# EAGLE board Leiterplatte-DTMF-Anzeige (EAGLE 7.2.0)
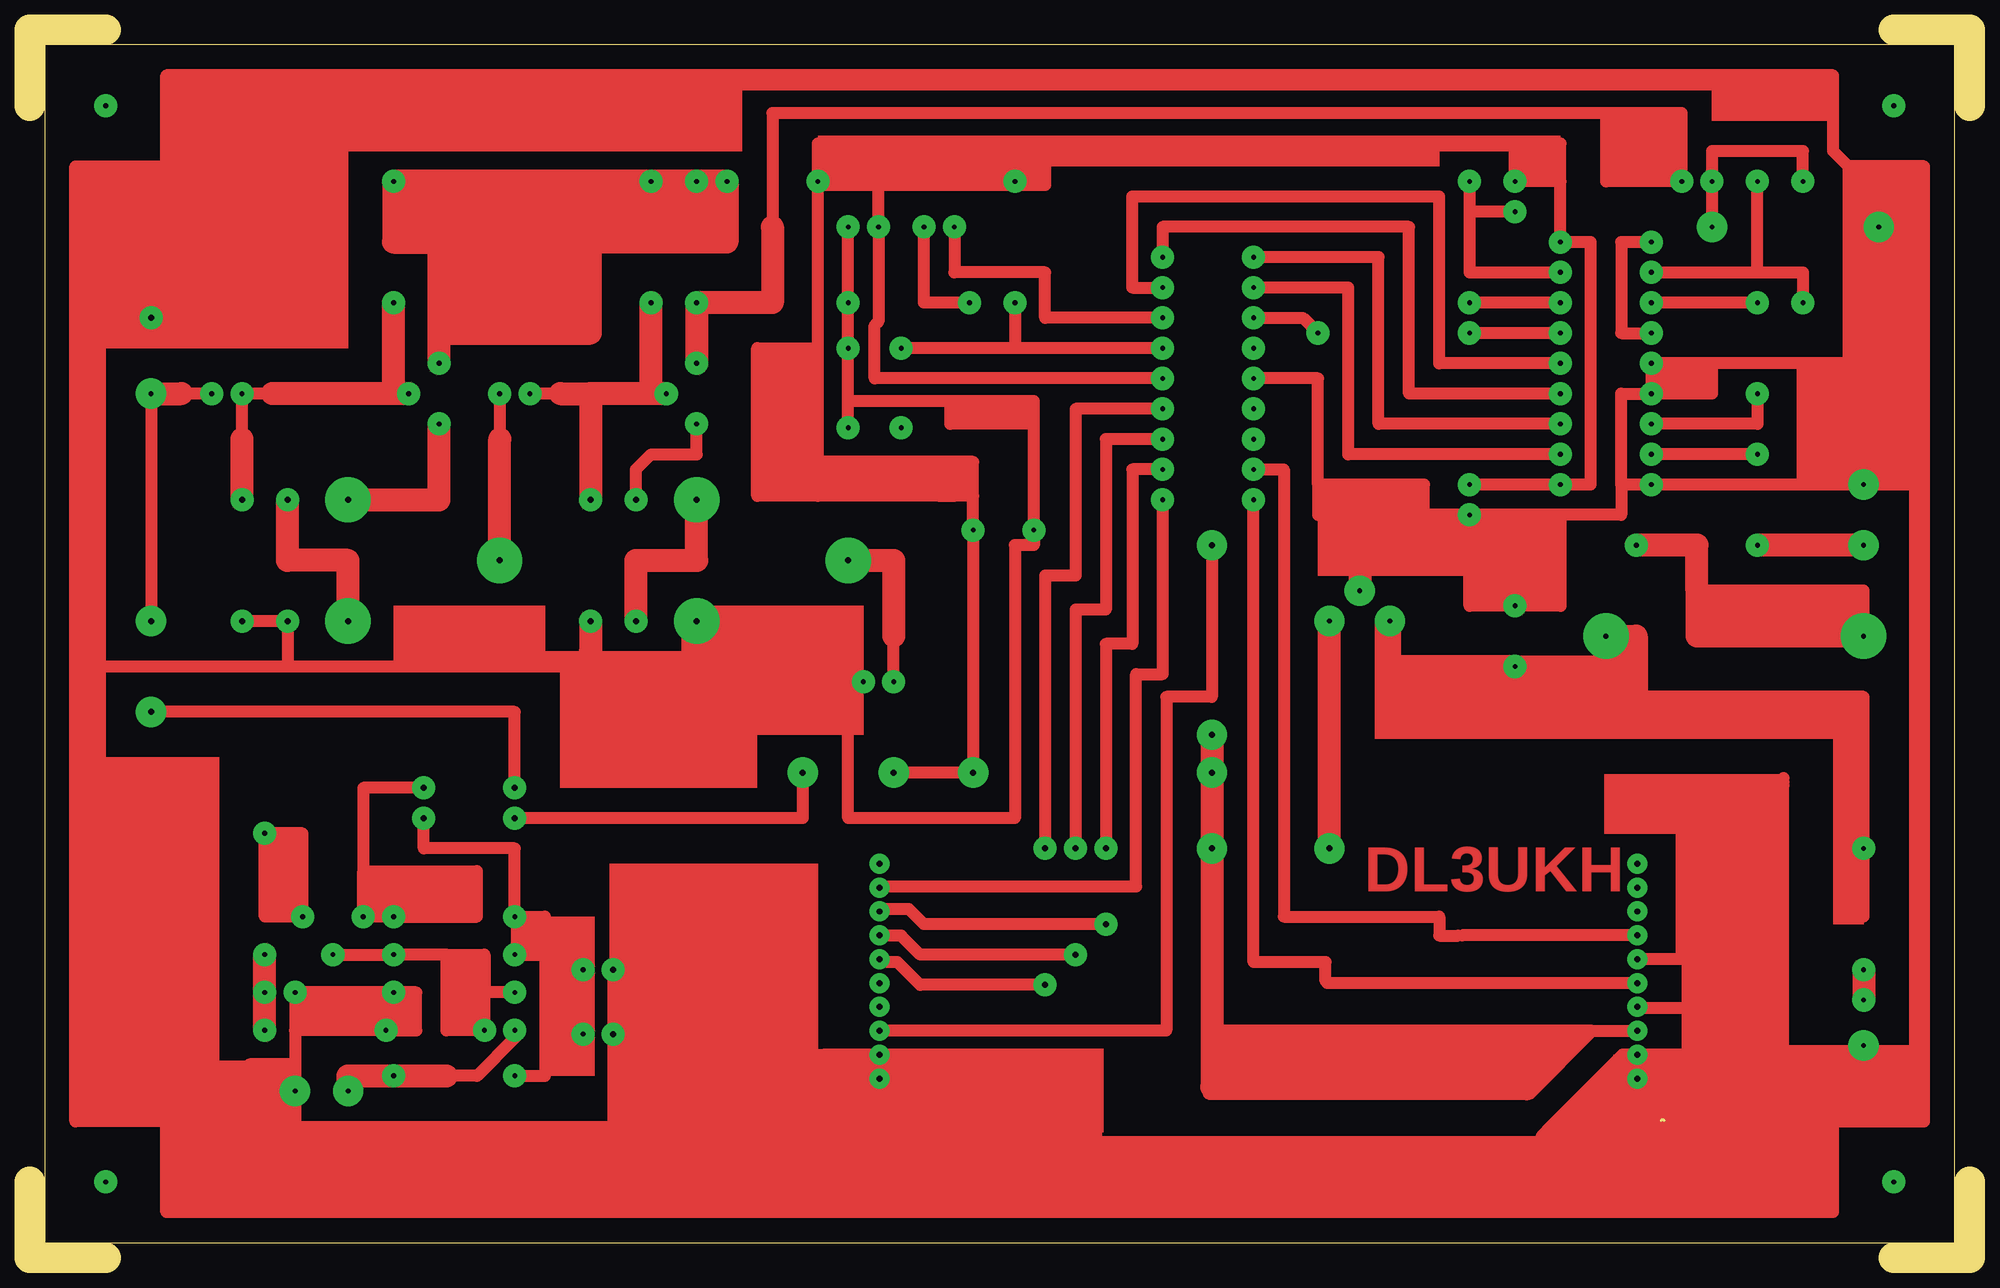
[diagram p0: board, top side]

Size 162.56 x 102.87 mm. Coordinates in mm from the lower left corner, seen from the top.
Outline: 0,96.52 0,102.87 6.35,102.87
Outline: 0,6.35 0,0 6.35,0
Outline: 156.21,0 162.56,0 162.56,6.35
Outline: 162.56,96.52 162.56,102.87 156.21,102.87
Outline: 136.95,11.5 136.7,11.5
Outline: 1.27,101.6 1.27,1.27 161.29,1.27 161.29,101.6 1.27,101.6
Copper layers (1*16): Top 0.035mm / dielectric 1.5mm / Bottom 0.035mm
Design rules "default": minimum track width 10mil, minimum drill 24mil, track to track 8mil, track to pad 8mil, pad to pad 8mil, via to via 8mil, smd to smd 8mil, copper to edge 40mil, drill to drill 8mil, minimum pad ring 10mil, minimum via ring 8mil, stop-mask expansion 4mil, vias tented up to drill 0mil, thermal gap 10mil

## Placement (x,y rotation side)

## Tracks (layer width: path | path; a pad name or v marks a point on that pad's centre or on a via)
S$1  (via drill 0.4 pad 1.93)
  other vias: 6.35,6.35
S$2  (via drill 0.4 pad 1.93)
  other vias: 6.35,96.52
S$3  (via drill 0.4 pad 1.93)
  other vias: 156.21,6.35
S$4  (via drill 0.4 pad 1.93)
  other vias: 156.21,96.52
S$5  (via drill 0.4 pad 1.93)
  other vias: 55.88,90.17
S$6  (via drill 0.4 pad 1.93)
  Top 1.016: v94.93,81.28 92.39,81.28 92.39,88.9 118.11,88.9 118.11,74.93 v128.27,74.93
S$7  (via drill 0.4 pad 1.93)
  Top 1.016: v82.55,90.17 81.28,93.03
S$8  (via drill 0.4 pad 1.93)
  Top 1.016: v94.93,76.2 82.55,76.2 | v82.55,80.01 82.55,76.2 | 82.55,76.2 v73.02,76.2 | v78.74,80.01 74.93,80.01 v74.93,86.36 | v94.93,78.74 85.09,78.74 85.09,82.55 77.47,82.55 v77.47,86.36
S$9  (via drill 0.4 pad 1.93)
  Top 1.016: 71.12,93.34 v71.12,86.36 71.12,78.42 70.8,78.1 70.8,73.66 v94.93,73.66
S$10  (via drill 0.4 pad 1.93, 0.4 pad 2.54)
  Top 1.016: v102.55,73.66 107.95,73.66 107.95,64.77 | 107.95,64.77 107.95,62.23 114.3,62.23 | 107.95,64.77 116.84,64.77 116.84,62.23 | 114.3,62.23 111.44,58.74 | 116.84,62.23 114.3,62.23 | v120.65,62.23 116.84,62.23 | v120.65,62.23 120.65,54.61 128.27,54.61 128.27,62.23 | 124.46,62.23 v120.65,62.23 | 124.46,62.23 124.46,58.42 | 128.27,62.23 124.46,62.23 | 128.27,62.23 133.35,62.23 133.35,64.77 | v135.89,72.39 133.35,72.39 133.35,64.77 | v135.89,72.39 140.97,72.39 140.97,74.93 | v135.89,72.39 v135.89,74.93 140.97,74.93 | 133.35,64.77 v135.89,64.77 148.59,64.77 | 148.59,64.77 148.59,74.93 | 152.4,74.93 148.59,74.93 | 152.4,74.93 154.94,74.93 | 148.59,74.93 140.97,74.93 | 152.4,91.44 151.13,92.71 151.13,99.06 11.43,99.06 11.43,91.44 3.81,91.44 3.81,50.8 | 152.4,91.44 152.4,74.93 | 152.4,64.77 148.59,64.77 | 152.4,64.77 152.4,74.93 | 152.4,64.77 v153.67,64.77 158.75,64.77 | 152.4,91.44 158.75,91.44 158.75,64.77 | 3.81,50.8 5.08,50.8 | 3.81,50.8 3.81,11.43 11.43,11.43 11.43,3.81 151.13,3.81 151.13,11.43 158.75,11.43 158.75,64.77
  Top 1.93: 111.44,58.74 v111.44,55.88 | 124.46,58.42 v124.46,54.61
S$11  (via drill 0.4 pad 1.93)
  other vias: 73.02,69.53
S$12  (via drill 0.4 pad 1.93)
  other vias: 102.55,68.58
S$13  (via drill 0.4 pad 1.93)
  other vias: 102.55,71.12
S$14  (via drill 0.4 pad 1.93)
  Top 1.016: 62.23,86.36 62.23,95.88 132.08,95.88 | 132.08,95.88 138.43,95.88 v138.43,90.17 132.08,90.17 132.08,95.88
  Top 1.93: v55.88,74.93 v55.88,80.01 62.23,80.01 62.23,86.36
S$15  (via drill 0.4 pad 1.93)
  Top 1.016: v68.58,86.36 v68.58,80.01 68.58,71.75 | v68.58,69.53 68.58,71.75 | 77.15,71.75 84.14,71.75 84.14,69.85 | 77.15,71.75 68.58,71.75 | 84.14,69.85 v84.14,60.96 84.14,59.69 82.55,59.69 82.55,36.83 68.58,36.83 68.58,44.45 | 84.14,69.85 77.15,69.85 77.15,71.75
S$16  (via drill 0.4 pad 2.54)
  other vias: 154.94,86.36
S$17  (via drill 0.4 pad 1.93)
  other vias: 68.58,76.2
S$18  (via drill 0.4 pad 1.93, 0.4 pad 3.81)
  Top 1.016: v153.67,52.07 153.67,55.88 139.7,55.88
  Top 1.93: v153.67,52.07 139.7,52.07 139.7,55.88 139.7,59.69 v134.62,59.69
S$19  (via drill 0.4 pad 1.93)
  Top 1.93: v153.67,24.13 v153.67,21.59
S$20  (via drill 0.5 pad 1.93)
  other vias: 10.16,78.74
S$21  (via drill 0.4 pad 1.93, 0.4 pad 2.54)
  Top 1.93: v153.67,59.69 v144.78,59.69
S$22  (via drill 0.4 pad 2.54)
  Top 1.93: 108.9,34.29 v108.9,53.34
S$23
  Top 1.016: 134.62,20.95 139.38,20.95
S$24  (via drill 0.4 pad 1.93, 0.4 pad 2.54)
  Top 1.016: v29.84,19.05 30.48,19.05 v30.48,22.22 | v30.48,22.22 v22.22,22.22 22.22,19.05 | v29.84,19.05 32.38,19.05 32.38,22.22 v30.48,22.22 | 22.22,19.05 v22.22,13.97 | v29.84,19.05 22.22,19.05 | v22.22,13.97 22.22,11.43 | 22.22,11.43 22.22,10.16 | 22.22,11.43 18.41,11.43 | 18.41,11.43 18.41,10.16 21.91,10.16 | v22.22,13.97 22.22,16.19 18.41,16.19 18.41,11.43
S$25  (via drill 0.4 pad 1.93)
  other vias: 102.55,66.04
S$26  (via drill 0.5 pad 1.93, 0.5 pad 2.54)
  Top 1.016: v40.64,39.37 40.64,45.72 v10.16,45.72
S$27  (via drill 0.5 pad 1.68)
  other vias: 134.7,21
S$28  (via drill 0.5 pad 1.68)
  Top 1.016: v134.7,31 134.75,31 134.75,31.06
S$29  (via drill 0.4 pad 1.93)
  Top 1.016: 124.46,93.34 v124.46,90.17 128.27,90.17 | 128.27,90.17 128.27,93.34 | 128.27,90.17 v128.27,85.09 130.81,85.09 130.81,64.77 v128.27,64.77 v120.65,64.77
S$30  (via drill 0.5 pad 1.68)
  Top 1.016: 71.35,31.07 71.35,31 v71.2,31
S$31  (via drill 0.5 pad 1.68)
  Top 1.016: 71.39,28.85 71.39,29 v71.2,29
S$32  (via drill 0.4 pad 1.93, 0.4 pad 2.54, 0.5 pad 2.54)
  Top 1.016: v15.24,72.39 12.7,72.39 | v10.16,72.39 v10.16,53.34
  Top 1.93: v10.16,72.39 12.7,72.39
S$33  (via drill 0.4 pad 1.93, 0.5 pad 1.93)
  Top 1.016: v94.93,66.04 92.39,66.04 92.39,51.44 90.17,51.44 v90.17,34.29
S$34  (via drill 0.4 pad 1.93, 0.5 pad 1.93)
  Top 1.016: v94.93,68.58 90.17,68.58 90.17,54.29 87.63,54.29 v87.63,34.29
S$35  (via drill 0.4 pad 1.93, 0.5 pad 1.93)
  Top 1.016: v94.93,71.12 87.63,71.12 87.63,57.15 85.09,57.15 v85.09,34.29
S$36  (via drill 0.4 pad 2.54)
  other vias: 153.67,17.78
S$37  (via drill 0.5 pad 1.68)
  Top 1.016: 71.11,26.94 71.11,27 v71.2,27
S$38  (via drill 0.5 pad 1.68)
  Top 1.016: 71.15,25.04 71.15,25 v71.2,25
S$39  (via drill 0.4 pad 1.93, 0.5 pad 3.81)
  Top 1.016: v39.37,72.39 39.37,68.58
  Top 1.93: v39.37,58.42 39.37,68.58
S$40  (via drill 0.5 pad 1.68)
  Top 1.016: 71.17,33.03 71.17,32.93 71.2,32.93 v71.2,33.01
S$41
  Top 1.016: 102.55,66.04 105.09,66.04 105.09,28.57 118.11,28.57 118.11,26.99 119.7,26.99
S$42  (via drill 0.4 pad 1.93, 0.5 pad 1.93)
  Top 1.016: v50.8,63.5 50.8,66.04 52.07,67.31 55.88,67.31 v55.88,69.85
S$43  (via drill 0.5 pad 1.93, 0.5 pad 3.81)
  Top 1.93: v50.8,53.34 50.8,58.42 55.88,58.42 v55.88,63.5
S$44  (via drill 0.4 pad 1.93, 0.5 pad 1.93, 0.5 pad 3.81)
  Top 1.016: v69.85,48.26 67.31,48.26 66.04,49.53 55.88,49.53 | 55.88,50.8 55.88,49.53 | v17.78,53.34 v21.59,53.34 21.59,49.53 | 46.99,50.8 46.99,49.53 | 46.99,49.53 21.59,49.53 | 21.59,49.53 6.35,49.53 | 55.88,49.53 46.99,49.53
  Top 1.93: v55.88,53.34 55.88,50.8 | v46.99,53.34 46.99,50.8
S$45  (via drill 0.4 pad 1.93, 0.5 pad 3.81)
  Top 1.016: v72.39,48.26 72.39,52.07
  Top 1.93: v68.58,58.42 72.39,58.42 72.39,52.07
S$46  (via drill 0.4 pad 1.93, 0.5 pad 1.93)
  Top 1.016: 44.45,72.39 v41.91,72.39
  Top 1.93: v52.07,80.01 52.07,72.39 v53.34,72.39 46.99,72.39 | 44.45,72.39 46.99,72.39 | 46.99,72.39 v46.99,63.5
S$47  (via drill 0.5 pad 1.68)
  Top 1.016: 134.79,29.16 134.79,29 v134.7,29
S$48  (via drill 0.5 pad 1.68)
  Top 1.016: 109.29,16.15 109.29,16.25 98.77,13.75 125.7,13.75 130.95,19 v134.7,19
S$49  (via drill 0.5 pad 1.68)
  Top 1.016: 70.98,19.09 70.98,19 v71.2,19
S$50  (via drill 0.4 pad 1.93)
  Top 1.016: v135.89,82.55 144.78,82.55 | 144.78,82.55 v144.78,90.17 | 144.78,82.55 148.59,82.55 v148.59,80.01
S$51  (via drill 0.4 pad 1.93)
  Top 1.016: v135.89,85.09 133.35,85.09 133.35,77.47 v135.89,77.47
S$52  (via drill 0.4 pad 1.93, 0.5 pad 3.81)
  Top 1.93: v26.67,63.5 34.29,63.5 v34.29,69.85
S$53  (via drill 0.5 pad 1.68)
  other vias: 134.7,15
S$54  (via drill 0.5 pad 1.68)
  Top 1.016: v71.2,15 67.34,15
S$55  (via drill 0.5 pad 1.68)
  Top 1.016: v134.7,33.01 134.39,33.01 134.39,32.97
S$56  (via drill 0.5 pad 1.93, 0.5 pad 3.81)
  Top 1.93: v26.67,53.34 26.67,58.42 21.59,58.42 v21.59,63.5
S$59
  Top 1.016: 147,10.48 147,9.84 126.68,9.84 | 126.68,9.84 126.68,10.16 128.91,12.38 | 126.68,9.84 126.68,4.13
S$60  (via drill 0.5 pad 2.54)
  other vias: 108.9,34.29
S$61  (via drill 0.5 pad 2.54)
  Top 1.93: v99.06,43.82 v99.06,40.64 v99.06,34.29 99.06,14.29
S$62
  Top 1.016: 125.41,13.65 125.41,13.97
S$63  (via drill 0.5 pad 1.68)
  other vias: 134.7,21
S$64  (via drill 0.5 pad 1.68)
  other vias: 134.7,25
S$65  (via drill 0.5 pad 1.68)
  Top 1.016: v71.2,17 67.34,17
S$66  (via drill 0.5 pad 1.68)
  other vias: 71.2,21
S$67  (via drill 0.5 pad 1.68)
  other vias: 71.2,23
S$68  (via drill 0.4 pad 1.93, 0.5 pad 1.93)
  Top 1.016: 20.32,72.39 v17.78,72.39 17.78,68.58
  Top 1.93: 30.48,72.39 v30.48,80.01 | 30.48,72.39 20.32,72.39 | v31.75,72.39 30.48,72.39 | v17.78,63.5 17.78,68.58
S$69  (via drill 0.5 pad 1.68)
  Top 1.016: v134.7,31 134.75,31 134.75,31.06
S$70  (via drill 0.5 pad 1.68)
  Top 1.016: 71.03,31.07 71.35,31 v71.2,31
S$71  (via drill 0.5 pad 1.68)
  Top 1.016: 71.07,28.85 71.07,29 v71.2,29
S$72  (via drill 0.5 pad 1.68)
  Top 1.016: 71.11,26.94 71.11,27 v71.2,27
S$73  (via drill 0.5 pad 1.68)
  Top 1.016: 71.15,25.04 71.15,25 v71.2,25
S$74  (via drill 0.5 pad 1.68)
  Top 1.016: 71.17,33.03 71.17,32.93 71.2,32.93 v71.2,33.01
S$75  (via drill 0.5 pad 1.68)
  Top 1.016: 134.79,29.16 134.79,29 v134.7,29
S$76  (via drill 0.5 pad 1.68)
  Top 1.016: 109.29,16.15 109.29,16.25 103.85,13.75 109.45,13.75 | 109.45,13.75 125.7,13.75 130.95,19 | 130.95,19 v134.7,19 | 130.95,19 109.45,19 109.45,13.75
S$77  (via drill 0.5 pad 1.68)
  Top 1.016: 71.3,19.09 71.3,19 v71.2,19
S$78  (via drill 0.5 pad 1.68)
  Top 1.016: v71.2,15 67.34,15
S$79  (via drill 0.5 pad 1.68)
  Top 1.016: v134.7,33.01 v134.71,33.01 134.71,32.97
S$82  (via drill 0.5 pad 1.68)
  other vias: 134.7,23
S$83  (via drill 0.5 pad 1.68)
  other vias: 134.7,23 134.7,23
S$84  (via drill 0.5 pad 1.68)
  other vias: 134.7,27
S$85  (via drill 0.5 pad 2.54)
  Top 1.016: v99.06,59.69 99.06,46.99 95.25,46.99 95.25,19.05 71.12,19.05
S$86  (via drill 0.4 pad 1.93)
  Top 1.016: 71.12,31.11 92.71,31.11 92.71,48.9 94.93,48.9 v94.93,63.5
S$87  (via drill 0.5 pad 1.93)
  Top 1.016: v90.17,27.94 74.93,27.94 73.66,29.21 71.12,29.21
S$88  (via drill 0.5 pad 1.93)
  Top 1.016: v48.89,24.13 48.89,4.13
S$89  (via drill 0.4 pad 1.68)
  Top 1.016: v134.7,25 134.73,25 134.73,25.34 134.83,25.03
  other vias: 134.7,21
S$90  (via drill 0.4 pad 1.68)
  Top 1.016: v71.2,17 67.97,17
S$91  (via drill 0.4 pad 1.68)
  other vias: 71.2,21
S$92  (via drill 0.4 pad 1.68)
  other vias: 71.2,23
S$93  (via drill 0.4 pad 1.68)
  Top 1.016: v134.7,31 134.75,31 134.75,31.06
S$94  (via drill 0.4 pad 1.68)
  Top 1.016: 71.03,31.07 71.35,31 v71.2,31
S$95  (via drill 0.4 pad 1.68)
  Top 1.016: 71.39,28.85 71.39,29 v71.2,29
S$96  (via drill 0.4 pad 1.68)
  Top 1.016: 71.11,26.94 71.11,27 v71.2,27
S$97  (via drill 0.4 pad 1.68)
  Top 1.016: 71.15,25.04 71.47,25 v71.2,25
S$98  (via drill 0.4 pad 1.68)
  Top 1.016: 71.17,33.03 71.17,32.93 71.2,32.93 v71.2,33.01
S$99  (via drill 0.4 pad 1.68)
  Top 1.016: 134.79,29.16 134.79,29 v134.7,29
S$100  (via drill 0.4 pad 1.68)
  Top 1.016: 109.29,16.15 109.61,16.25 102.58,13.75 109.45,13.75 | 109.45,13.75 125.7,13.75 130.95,19 | 130.95,19 v134.7,19 | 130.95,19 109.45,19 109.45,13.75
S$101  (via drill 0.4 pad 1.93)
  Top 1.93: 34.29,90.17 v52.07,90.17 v58.42,90.17 58.42,85.09 35.56,85.09 34.29,85.09 | 34.29,90.17 v30.48,90.17 30.48,85.09 34.29,85.09 | v34.29,74.93 34.29,77.47 | 34.29,77.47 34.29,85.09 | 34.29,85.09 34.29,90.17 | 34.29,77.47 46.99,77.47 46.99,86.36
S$102  (via drill 0.4 pad 1.93)
  Top 1.016: v128.27,80.01 v120.65,80.01
S$103  (via drill 0.4 pad 1.93)
  Top 1.016: v128.27,77.47 v120.65,77.47
S$104  (via drill 0.4 pad 1.68)
  Top 1.016: 71.3,19.09 71.3,19 v71.2,19
S$105  (via drill 0.4 pad 1.93)
  Top 1.016: v128.27,72.39 115.57,72.39 115.57,86.36 94.93,86.36 v94.93,83.82
S$106  (via drill 0.4 pad 1.93)
  Top 1.016: v128.27,69.85 113.03,69.85 113.03,83.82 v102.55,83.82
S$107  (via drill 0.4 pad 1.93)
  Top 1.016: v128.27,67.31 110.49,67.31 110.49,81.28 v102.55,81.28
S$108  (via drill 0.4 pad 1.93)
  Top 1.016: v102.55,78.74 106.68,78.74 v107.95,77.47
S$109  (via drill 0.4 pad 1.68)
  Top 1.016: v71.2,15 67.34,15
S$110  (via drill 0.4 pad 1.93)
  other vias: 102.55,76.2
S$111  (via drill 0.4 pad 1.68)
  Top 1.016: v134.7,33.01 v134.71,33.01 134.71,32.97
S$113  (via drill 0.4 pad 1.68)
  Top 1.016: v134.7,23 108.7,23 108.7,23.12
S$114  (via drill 0.4 pad 1.68)
  Top 1.016: v134.7,23 126.45,23
S$115  (via drill 0.4 pad 1.93)
  Top 1.016: v120.65,90.17 120.65,87.63 | 120.65,87.63 120.65,82.55 v128.27,82.55 | v124.46,87.63 120.65,87.63
S$116  (via drill 0.4 pad 1.68)
  Top 1.016: v134.7,27 120.02,27
S$117  (via drill 0.4 pad 1.93)
  Top 1.016: 46.35,26.99 v46.35,24.13 v46.35,18.73 | 46.35,15.88 v46.35,18.73 | v46.35,18.73 46.35,25.4
S$118  (via drill 0.4 pad 1.93)
  Top 1.016: v144.78,67.31 v135.89,67.31
S$119  (via drill 0.4 pad 1.93)
  Top 1.016: v144.78,72.39 144.78,69.85 v135.89,69.85
S$120  (via drill 0.4 pad 1.93)
  Top 1.016: v144.78,80.01 v135.89,80.01
S$121  (via drill 0.4 pad 1.68)
  Top 1.016: 128.45,11 132.45,15 v134.7,15 v134.7,17 133.45,17 127.2,10.75
S$123  (via drill 0.4 pad 1.93, 0.4 pad 2.54)
  Top 1.016: v148.59,90.17 148.59,92.71 140.97,92.71 v140.97,90.17 v140.97,86.36
S$124  (via drill 0.5 pad 1.68)
  Top 1.016: 128.45,11 132.45,15 v134.7,15 v134.7,17 133.45,17 127.2,10.75
S$125  (via drill 0.5 pad 1.93)
  Top 1.016: v87.63,25.4 74.61,25.4 73.02,26.99 71.12,26.99
S$126  (via drill 0.5 pad 1.93)
  Top 1.016: v85.09,22.86 74.61,22.86 72.71,24.77 71.12,24.77
S$127  (via drill 0.4 pad 1.93)
  Top 1.016: 66.04,93.34 v66.04,90.17 66.04,89.85 | 66.04,76.2 66.04,89.85 | 66.04,63.82 66.04,66.67 | 66.04,66.67 66.04,76.2 | 66.04,76.2 60.96,76.2 60.96,63.82 76.2,63.82 | 76.2,63.82 77.47,63.82 | 85.09,91.44 85.09,89.85 66.04,89.85 | 76.2,63.82 76.2,66.67 | 76.2,66.67 66.04,66.67 | 77.47,63.82 77.47,66.67 | 77.47,66.67 76.2,66.67 | 79.06,63.82 v79.06,60.96 79.06,40.64 | 79.06,63.82 77.47,63.82 | 79.06,63.82 79.06,66.67 77.47,66.67
S$128  (via drill 0.5 pad 2.54)
  Top 1.016: v79.06,40.64 v72.39,40.64
S$129  (via drill 0.4 pad 1.68)
  Top 1.016: 134.63,21 v134.7,21 | 146.7,25 145.95,25 | 145.95,25 134.73,25 | v134.7,25 134.73,25 | 134.73,25 134.73,25.03 134.83,25.03 | 128.45,11 132.45,15 v134.7,15 | 127.2,10.75 133.45,17 v134.7,17 | v134.7,15 139.7,15 | v134.7,17 v134.7,15 | 138.95,17 v134.7,17 | 138.95,17 145.95,17 | 145.95,17 146.45,17 | 138.95,10.39 138.95,17 | 145.95,25 145.95,17
S$130  (via drill 0.4 pad 1.93, 0.4 pad 2.54, 0.4 pad 3.81)
  Top 1.016: v124.46,49.53 124.46,45.72 151.13,45.72 151.13,46.99 | 151.13,46.99 133.35,46.99 | 151.13,46.99 153.67,46.99 v153.67,34.29 | v153.67,34.29 152.4,34.29 | 153.67,30.48 v153.67,34.29 | 153.67,30.48 151.76,30.48 | 153.67,28.57 153.67,30.48
  Top 1.93: 134.62,46.99 134.62,52.07 v132.08,52.07 132.08,49.53 v124.46,49.53 113.98,49.53 | 113.98,49.53 v113.98,53.34 | 113.98,49.53 113.98,46.99
S$131  (via drill 0.4 pad 1.68)
  Top 1.016: v71.2,17 67.34,17
S$132  (via drill 0.4 pad 1.68)
  other vias: 71.2,21
S$133  (via drill 0.4 pad 1.68)
  other vias: 71.2,23
S$134  (via drill 0.4 pad 1.68)
  Top 1.016: v134.7,31 134.75,31 134.75,31.06
S$135  (via drill 0.4 pad 1.68)
  Top 1.016: 71.35,31.07 71.35,31 v71.2,31
S$136  (via drill 0.4 pad 1.68)
  Top 1.016: 71.39,28.85 71.07,29 v71.2,29
S$137  (via drill 0.4 pad 1.68)
  Top 1.016: 71.11,26.94 71.11,27 v71.2,27
S$138  (via drill 0.4 pad 1.68)
  Top 1.016: 71.15,25.04 71.15,25 v71.2,25
S$139  (via drill 0.4 pad 1.68)
  Top 1.016: 71.17,33.03 71.17,33.24 71.2,33.24 v71.2,33.01
S$140  (via drill 0.4 pad 1.68)
  Top 1.016: 134.79,29.16 134.79,29 v134.7,29
S$141  (via drill 0.4 pad 1.68)
  Top 1.016: 109.29,16.15 108.66,16.25 103.53,13.75 109.45,13.75 | 109.45,13.75 125.7,13.75 130.95,19 | 130.95,19 v134.7,19 | 130.95,19 98.98,19 109.45,13.75
S$142  (via drill 0.4 pad 1.68)
  Top 1.016: 71.3,19.09 71.3,19 v71.2,19
S$143  (via drill 0.4 pad 1.68)
  Top 1.016: v71.2,15 67.97,15
S$144  (via drill 0.4 pad 1.68)
  Top 1.016: v134.7,33.01 v134.71,33.01 134.71,32.97
S$146  (via drill 0.4 pad 1.68)
  Top 1.016: v134.7,23 109.02,23 108.7,23.12
S$147  (via drill 0.4 pad 1.68)
  Top 1.016: v134.7,23 126.45,23
S$148  (via drill 0.4 pad 1.68)
  other vias: 134.7,27
S$149  (via drill 0.4 pad 1.93)
  Top 1.016: v22.86,28.57 22.86,35.56 v19.69,35.56 19.69,28.57 v22.86,28.57
S$151  (via drill 0.4 pad 1.93)
  Top 1.016: v19.69,25.4 v19.69,22.22 v19.69,19.05
  Top 1.93: v19.69,19.05 v19.69,25.4
S$152
  Top 1.016: 146.95,10.46 146.95,39.55
S$153
  Top 1.016: 146.95,10.46 146.95,39.87
S$154
  Top 1.016: 146.95,10.78 146.95,40.19
S$155  (via drill 0.4 pad 1.93)
  Top 1.016: 108.58,23.18 108.58,24.77 102.55,24.77 v102.55,63.5
S$156  (via drill 0.4 pad 1.93)
  Top 1.016: v40.64,22.22 38.1,22.22 | 38.1,22.22 34.92,22.22 | 34.92,22.22 34.92,25.4 | v25.4,25.4 v30.48,25.4 34.92,25.4 | 34.92,22.22 34.92,19.05 v38.1,19.05 38.1,22.22 | 34.92,25.4 38.1,25.4 38.1,22.22
S$157  (via drill 0.4 pad 1.93, 0.4 pad 2.54)
  Top 1.016: v40.64,19.05 40.64,18.41 37.46,15.24 34.92,15.24 v30.48,15.24 26.67,15.24
  Top 1.93: v26.67,13.97 26.67,15.24 34.92,15.24
S$158  (via drill 0.5 pad 1.93)
  other vias: 48.89,18.73
S$160  (via drill 0.4 pad 1.93, 0.5 pad 1.93)
  Top 1.016: 43.18,25.4 43.18,28.57 v40.64,28.57 40.64,34.29 33.02,34.29 v33.02,36.83 | 43.18,25.4 43.18,15.24 v40.64,15.24 | v40.64,25.4 43.18,25.4
S$161  (via drill 0.4 pad 1.93, 0.5 pad 1.93)
  Top 1.016: 27.94,32.38 v27.94,28.57 v30.48,28.57 37.46,28.57 37.46,32.38 27.94,32.38 | v33.02,39.37 27.94,39.37 27.94,32.38
S$163  (via drill 0.5 pad 1.93, 0.5 pad 2.54)
  Top 1.016: v64.77,40.64 64.77,36.83 v40.64,36.83
(copper drawn outside any net)
  shapes: Top area x97

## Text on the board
Top: DL3UKH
